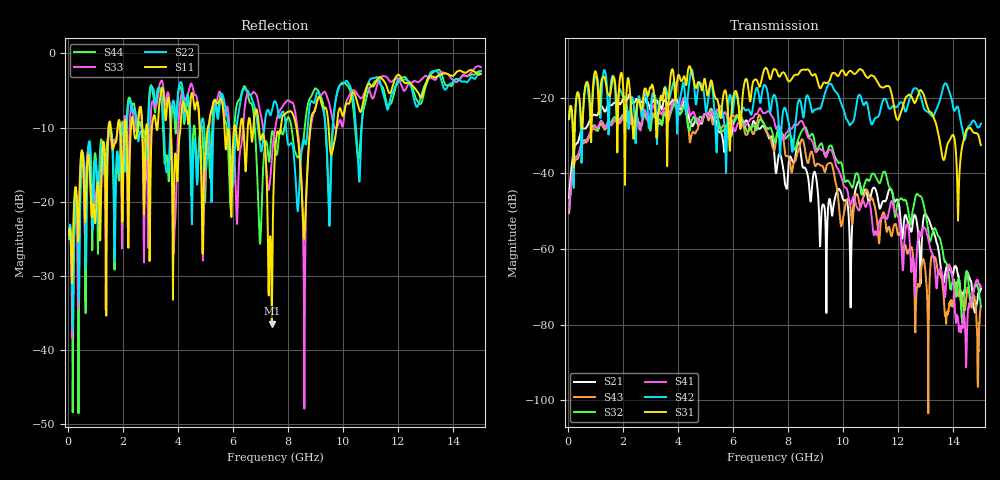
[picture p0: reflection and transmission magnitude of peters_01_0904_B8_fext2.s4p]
# MHZ S RI R 50.00
! FREQ  S11  S12  S13  S14
!  S21  S22  S23  S24
!  S31  S32  S33  S34
!  S41  S42  S43  S44
!  REAL  IMAG  REAL  IMAG  REAL  IMAG  REAL  IMAG
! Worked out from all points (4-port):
!   1496 points, 50 MHz to 15 GHz, reference 50 ohm
!   strongest paths, dB at 50 MHz, 3.79 GHz, 7.53 GHz, 11.27 GHz, 15 GHz:
!     S31: -25.6, -12.4, -12.4, -16.1, -32.5
!     S42: -25.6, -17.2, -19.5, -25.0, -26.8
!     S41: -49.7, -21.5, -27.3, -54.5, -69.9
!     S32: -49.9, -22.9, -31.8, -42.1, -75.0
!     S43: -50.5, -22.4, -33.0, -55.9, -75.1
!     S21: -46.5, -20.7, -38.0, -47.2, -70.5
!   lowest |S11| = -36.5 dB at 7.41 GHz (marker M1), VSWR 1.03, Z = 51.5 + j0.182 ohm
!   |S11| at or under -10 dB: start of sweep to 1.487 GHz; 6.944 GHz to 7.736 GHz (791.8 MHz wide, 10.8 % of centre); 8.3 GHz to 8.803 GHz (502.7 MHz wide, 5.88 % of centre)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
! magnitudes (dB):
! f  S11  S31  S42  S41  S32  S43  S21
! 50 MHz  -24.4  -25.6  -25.6  -49.7  -49.9  -50.5  -46.5
! 2.23 GHz  -17.9  -16.0  -27.0  -24.1  -23.7  -25.7  -19.1
! 6.85 GHz  -7.5  -15.2  -17.4  -24.3  -28.5  -27.1  -27.7
! 7.41 GHz  -36.5  -13.7  -21.1  -24.9  -28.7  -32.3  -30.3
! 7.88 GHz  -8.2  -13.5  -22.6  -30.1  -30.7  -34.2  -42.3
! 8.59 GHz  -24.9  -12.5  -23.7  -27.5  -27.8  -32.6  -38.4
! 15 GHz  -2.8  -32.5  -26.8  -69.9  -75.0  -75.1  -70.5
